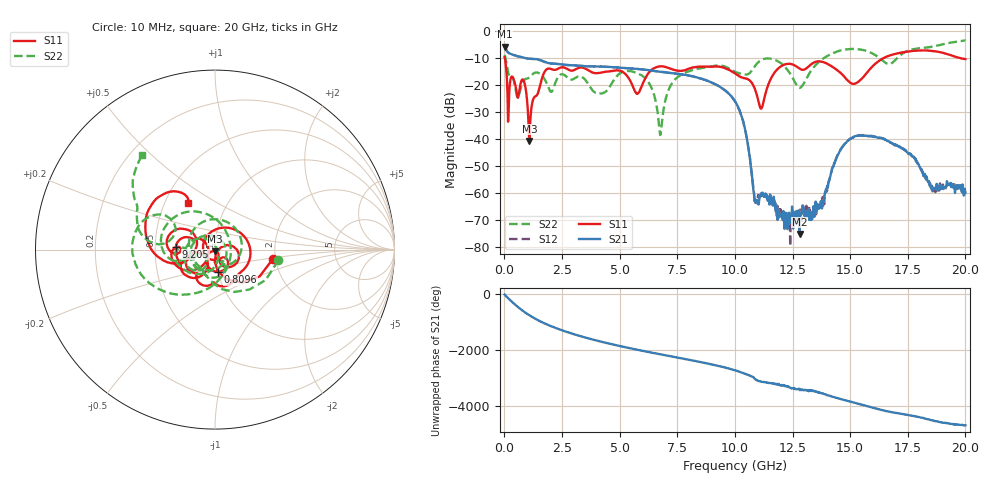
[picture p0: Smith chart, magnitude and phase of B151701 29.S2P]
!  2-Port S-parameters saved by WinCal
! VAR MeasName=S-Parameters (CALIBRATED_DATA) read from VNA (N5244A)
! VAR MeasDate=2015-12-24 19:11:29
! VAR NAME=B151701 29
! VAR FILENAME=B151701 29.S2P
! VAR DATE=2015-12-24 19:11:29
! VAR PHYS_PORTS=1,3
# Hz S DB R 50
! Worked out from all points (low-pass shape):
!   801 points, 10 MHz to 20 GHz, reference 50 ohm
!   highest |S21| = -5.89 dB at 10 MHz (marker M1); lowest = -75.2 dB at 12.8 GHz (marker M2)
!   |S21| within 3 dB of the highest: start of sweep to 372.9 MHz
!   lowest |S11| = -40.8 dB at 1.084 GHz (marker M3), VSWR 1.02, Z = 50 - j0.916 ohm
!   |S11| at or under -10 dB: 16.22 MHz to 16.48 GHz (16.46 GHz wide, 200 % of centre); 19.72 GHz to end of sweep
!   |S22| runs from -38.6 to -3.6 dB; largest |S21 - S12| = 0.0025
!   S11 on the Smith chart (normalised r, x): 10 MHz: 1.93, -0.23; 809.6 MHz: 1.00, -0.25; 9.205 GHz: 0.64, +0.02; 20 GHz: 0.65, +0.37
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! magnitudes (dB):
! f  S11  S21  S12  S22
! 10 MHz  -9.7  -5.9  -5.9  -8.9
! 209.9 MHz  -23.0  -8.3  -8.3  -16.7
! 809.6 MHz  -18.1  -9.9  -9.9  -18.7
! 1.084 GHz  -40.8  -10.4  -10.3  -17.3
! 1.809 GHz  -14.4  -11.7  -11.7  -18.9
! 3.358 GHz  -13.6  -13.0  -13.0  -17.1
! 4.158 GHz  -15.5  -13.2  -13.2  -23.2
! 5.907 GHz  -21.5  -14.2  -14.2  -16.2
! 6.682 GHz  -13.2  -15.1  -15.1  -32.5
! 7.456 GHz  -14.6  -15.8  -15.8  -17.6
! 9.205 GHz  -13.2  -20.0  -20.0  -12.9
! 10.01 GHz  -15.7  -26.1  -26.1  -15.2
! 10.43 GHz  -17.5  -36.0  -36.0  -16.2
! 10.93 GHz  -23.1  -63.6  -62.6  -12.4
! 11.15 GHz  -28.7  -60.2  -61.2  -10.8
! 11.85 GHz  -14.1  -70.0  -64.8  -11.2
! 12.8 GHz  -14.0  -75.2  -67.3  -21.1
! 13.35 GHz  -12.1  -69.5  -69.7  -14.2
! 14.88 GHz  -18.2  -40.9  -40.8  -6.8
! 16.68 GHz  -9.2  -40.9  -41.0  -12.3
! 18.6 GHz  -7.5  -58.4  -57.7  -5.8
! 20 GHz  -10.5  -59.9  -60.6  -3.6
